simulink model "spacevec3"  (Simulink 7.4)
settings: Solver=ode45  StartTime=0.0  StopTime=10.0  RelTol=1e-3

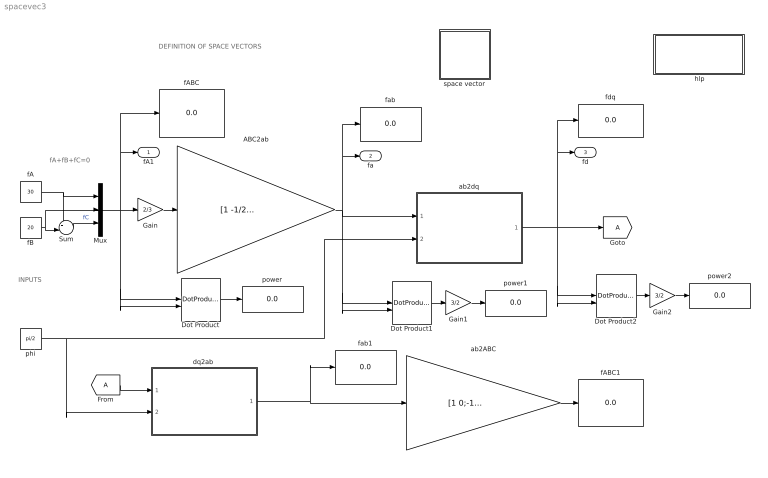
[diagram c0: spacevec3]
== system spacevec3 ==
  note: DEFINITION OF SPACE VECTORS
  note: fA+fB+fC=0
  note: INPUTS
  " hlp" : Subsystem
  ABC2ab : Gain  Gain=[1 -1/2 -1/2;0 sqrt(3)/2 -sqrt(3)/2]  Multiplication=Matrix(K*u)  ParameterDataType=sfix(16)  ParameterScaling=2^0  OutDataType=sfix(16)  OutScaling=2^0
  Dot Product : DotProduct  OutDataType=fixdt(1, 16)  OutScaling=2^-10
  Dot Product1 : DotProduct  OutDataType=fixdt(1, 16)  OutScaling=2^-10
  Dot Product2 : DotProduct  OutDataType=fixdt(1, 16)  OutScaling=2^-10
  Gain : Gain  Gain=2/3  ParameterDataType=sfix(16)  ParameterScaling=2^0  OutDataType=sfix(16)  OutScaling=2^0
  Gain1 : Gain  Gain=3/2  ParameterDataType=sfix(16)  ParameterScaling=2^0  OutDataType=sfix(16)  OutScaling=2^0
  Gain2 : Gain  Gain=3/2  ParameterDataType=sfix(16)  ParameterScaling=2^0  OutDataType=sfix(16)  OutScaling=2^0
  Mux : Mux  Inputs=3
  Sum : Sum  Inputs=--|  OutDataType=sfix(16)  OutScaling=2^0
  ab2ABC : Gain  Gain=[1 0;-1/2 sqrt(3)/2;-1/2 -sqrt(3)/2]  Multiplication=Matrix(K*u)  ParameterDataType=sfix(16)  ParameterScaling=2^0  OutDataType=sfix(16)  OutScaling=2^0
  ab2dq : Subsystem
  "dq2ab " : Subsystem
  fA : Constant  Value=30  OutDataType=sfix(16)  OutScaling=2^0
  fABC : Display
  fABC1 : Display
  fB : Constant  Value=20  OutDataType=sfix(16)  OutScaling=2^0
  fab : Display
  fab1 : Display
  fdq : Display
  phi : Constant  Value=pi/2  OutDataType=sfix(16)  OutScaling=2^0
  power : Display
  power1 : Display
  power2 : Display
  space vector : Subsystem
  fA1 : Outport
  fa : Outport  Port=2
  fd : Outport  Port=3
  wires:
  Mux/1 -> Dot Product/2, Dot Product/1, Gain/1, fABC/1, fA1/1
  ABC2ab/1 -> Dot Product1/2, Dot Product1/1, fab/1, fa/1, ab2dq/1(ab)
  ab2dq/1(dq) -> [A], fdq/1, fd/1, Dot Product2/2, Dot Product2/1
  Dot Product/1 -> power/1
  Dot Product1/1 -> Gain1/1
  Gain1/1 -> power1/1
  "dq2ab "/1(ab) -> ab2ABC/1, fab1/1
  ab2ABC/1 -> fABC1/1
  Gain/1 -> ABC2ab/1
  fA/1 -> Sum/1, Mux/1
  fB/1 -> Sum/2, Mux/2
  Sum/1 -> Mux/3  "fC"
  [A] -> "dq2ab "/1(dq)
  phi/1 -> ab2dq/2(phi), "dq2ab "/2(phi)
  Dot Product2/1 -> Gain2/1
  Gain2/1 -> power2/1

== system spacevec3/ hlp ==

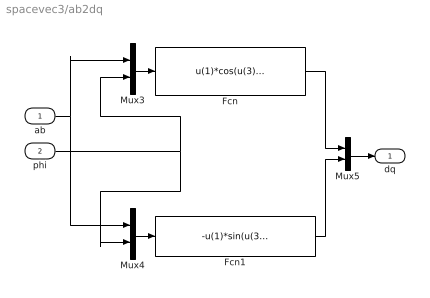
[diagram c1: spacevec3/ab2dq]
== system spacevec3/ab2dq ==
  ab : Inport  OutDataType=sfix(16)  OutScaling=2^0
  phi : Inport  Port=2  OutDataType=sfix(16)  OutScaling=2^0
  Fcn : Fcn  Expr=u(1)*cos(u(3))+u(2)*sin(u(3))
  Fcn1 : Fcn  Expr=-u(1)*sin(u(3))+u(2)*cos(u(3))
  Mux3 : Mux  Inputs=2
  Mux4 : Mux  Inputs=2
  Mux5 : Mux  Inputs=2
  dq : Outport
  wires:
  Mux3/1 -> Fcn/1
  Mux4/1 -> Fcn1/1
  ab/1 -> Mux3/1, Mux4/1
  phi/1 -> Mux3/2, Mux4/2
  Fcn1/1 -> Mux5/2
  Fcn/1 -> Mux5/1
  Mux5/1 -> dq/1

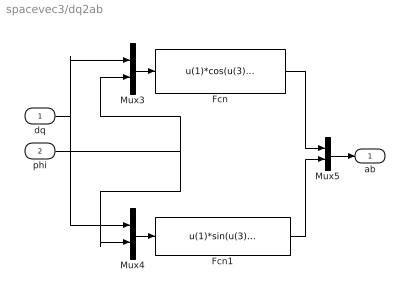
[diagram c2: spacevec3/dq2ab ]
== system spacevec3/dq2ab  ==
  dq : Inport  OutDataType=sfix(16)  OutScaling=2^0
  phi : Inport  Port=2  OutDataType=sfix(16)  OutScaling=2^0
  Fcn : Fcn  Expr=u(1)*cos(u(3))-u(2)*sin(u(3))
  Fcn1 : Fcn  Expr=u(1)*sin(u(3))+u(2)*cos(u(3))
  Mux3 : Mux  Inputs=2
  Mux4 : Mux  Inputs=2
  Mux5 : Mux  Inputs=2
  ab : Outport
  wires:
  Mux5/1 -> ab/1
  Fcn/1 -> Mux5/1
  Fcn1/1 -> Mux5/2
  phi/1 -> Mux4/2, Mux3/2
  dq/1 -> Mux4/1, Mux3/1
  Mux4/1 -> Fcn1/1
  Mux3/1 -> Fcn/1

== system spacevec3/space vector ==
